FUNCTION_BLOCK ServoDriver_DI(*伺服驱动器的数字量输入*)
VAR_INPUT

END_VAR
VAR_OUTPUT
END_VAR
VAR
	di_UDint AT%I*:			UDINT;(*数字量*)
	di_Uint AT%I*:			UINT;(*数字量*)
	ErrorCode AT%I*:		UDINT;(*伺服硬件错误号*)
	EL1008 AT%I*:           BYTE;
	EL1004 AT%I*:           BOOL;

	bHomeSenser:			BOOL;(*原点信号*)
	bLimitSenser_P:			BOOL;(*正向限位*)
	bLimitSenser_N:			BOOL;(*负向限位*)
	bHwError:					BOOL;(*硬件报警*)
END_VAR




	bHomeSenser 	:= di_UDint.2 OR di_Uint.2OR EL1004;	(*home=2, Plimit=1,Nlimit=0*)
	bLimitSenser_P 	:= di_UDint.1 OR di_Uint.4OR EL1008.0;
	bLimitSenser_N 	:= di_UDint.0 OR di_Uint.5OR EL1008.1;

IF errorcode=16#D012 OR errorcode=16#D013 THEN
	 bHwError			:= FALSE;
ELSE bHwError			:= TRUE; 
END_IF                                                       (* ErrorCode<>0;*)

END_FUNCTION_BLOCK
